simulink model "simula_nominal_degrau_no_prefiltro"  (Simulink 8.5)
settings: Solver=ode45  StartTime=0.0  StopTime=tf  RelTol=1e-3
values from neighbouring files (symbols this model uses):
  denF = [1 qsi2wn wn2]    [princi_JL_incerto_prefilt_2a_ordem.m]
  denK = [1/6 1]    [princi_JL_incerto_prefilt_2a_ordem.m]
  knom = r*kT/Ra/Jeq    [princi_JL_incerto_prefilt_2a_ordem.m]
  numF = [wn2]    [princi_JL_incerto_prefilt_2a_ordem.m]
  numK = 2.5    [princi_JL_incerto_prefilt_2a_ordem.m]
  pnom = feq/Jeq    [princi_JL_incerto_prefilt_2a_ordem.m]

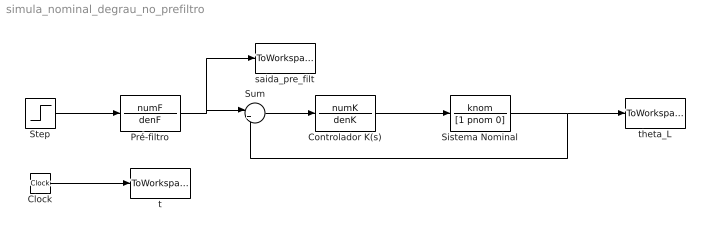
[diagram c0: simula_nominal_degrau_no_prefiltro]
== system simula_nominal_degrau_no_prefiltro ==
  Clock : Clock
  Controlador K(s) : TransferFcn  Numerator=numK  Denominator=denK
  Pré-filtro : TransferFcn  Numerator=numF  Denominator=denF
  Sistema Nominal : TransferFcn  Numerator=knom  Denominator=[1 pnom 0]
  Step : Step  Time=0  SampleTime=0
  Sum : Sum  Inputs=|+-
  saida_pre_filt : ToWorkspace  VariableName=saida_pre_filt  SampleTime=-1
  t : ToWorkspace  VariableName=t  SampleTime=-1
  theta_L : ToWorkspace  VariableName=theta_L_nom  SampleTime=-1
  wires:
  Sum/1 -> Controlador K(s)/1
  Pré-filtro/1 -> saida_pre_filt/1, Sum/1
  Clock/1 -> t/1
  Controlador K(s)/1 -> Sistema Nominal/1
  Sistema Nominal/1 -> Sum/2, theta_L/1
  Step/1 -> Pré-filtro/1
